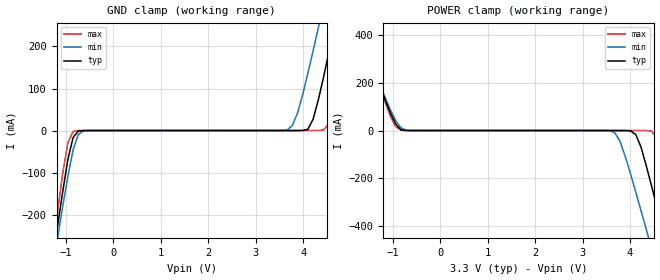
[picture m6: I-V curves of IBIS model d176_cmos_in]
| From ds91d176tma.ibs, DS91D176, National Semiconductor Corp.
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[Model]   d176_cmos_in
Model_type Input
Vinh=2.0
Vinl=0.8
|   Typ   Min   Max
C_comp   2.4pF   2.4pF   2.4pF
[Model Spec]
S_overshoot_high   3.3   3.0   3.6
S_overshoot_low   0.0   0.0   0.0
[Temperature Range]   25   85   -40
[Voltage Range]   3.3   3.0   3.6
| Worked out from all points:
|   GND clamp passes 1 mA (typ) near -0.71 V on its own axis
|   POWER clamp passes 1 mA (typ) near -0.75 V on its own axis
[GND Clamp]
-3.6V     -2.181A    -2.025A    -2.42A
-1.29V    -314mA     -334mA     -293mA
-1.18V    -229mA     -257mA     -196mA
-960mV    -68.6mA    -109mA     -29mA
-850mV    -16.4mA    -45.6mA    -2.22mA
-630mV    -40.1uA    -816uA     -3.6uA
3.66V     2.51uA     1.38mA     5.04uA
4.1V      3.04mA     137mA      5.04uA
4.32V     73.2mA     245mA      20.5uA
4.65V     244mA      415mA      59mA
4.98V     425mA      588mA      243mA
7.18V     1.672A     1.762A     1.577A
[POWER Clamp]
-3.58V    1.483A     1.408A     1.577A
-1.71V    425mA      415mA      438mA
-1.05V    73.2mA     85.6mA     59mA
-830mV    3.04mA     11.5mA     1.34mA
3.68V     -1.25uA    -9.28mA    -396nA
4.12V     -16.4mA    -257mA     -2.75uA
4.34V     -146mA     -412mA     -34.4uA
4.45V     -229mA     -491mA     -2.22mA
4.67V     -400mA     -650mA     -102mA
5V        -663mA     -890mA     -392mA
5.11V     -752mA     -971mA     -491mA
6.54V     -1.912A    -2.025A    -1.808A
